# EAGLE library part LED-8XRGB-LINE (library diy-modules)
8 LEDs RGB Line Display based on WS2812B More details about controlling WS2812B RGB LEDs are available here: https://learn.sparkfun.com/tutorials/ws2812-breakout-hookup-guide Click here to find device on ebay.com
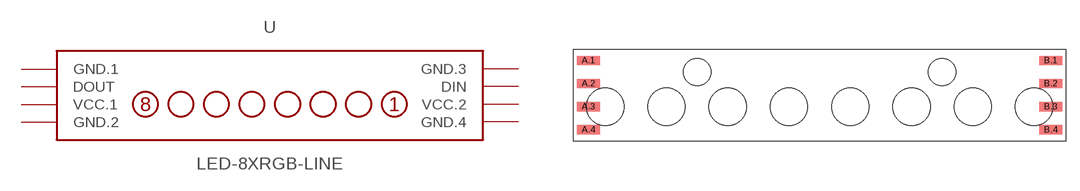
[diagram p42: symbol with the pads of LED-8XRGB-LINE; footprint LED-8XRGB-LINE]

Designator prefix -

## LED-8XRGB-LINE  [LED-8XRGB-LINE]
A.1  GND.1  pwr
A.2  DOUT  out
A.3  VCC.1  pwr
A.4  GND.2  pwr
B.1  GND.3  pwr
B.2  DIN  in
B.3  VCC.2  pwr
B.4  GND.4  pwr

## Footprint LED-8XRGB-LINE (pad centres in mm)
8 LEDs RGB Line Display based on WS2812B
smd 2.54 x 1.016: A.1 -25.4,3.81; A.2 -25.4,1.27; A.3 -25.4,-1.27; A.4 -25.4,-3.81; B.1 25.4,3.81; B.2 25.4,1.27; B.3 25.4,-1.27; B.4 25.4,-3.81
hole 3 at -13.462,2.54
hole 3 at 13.462,2.54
